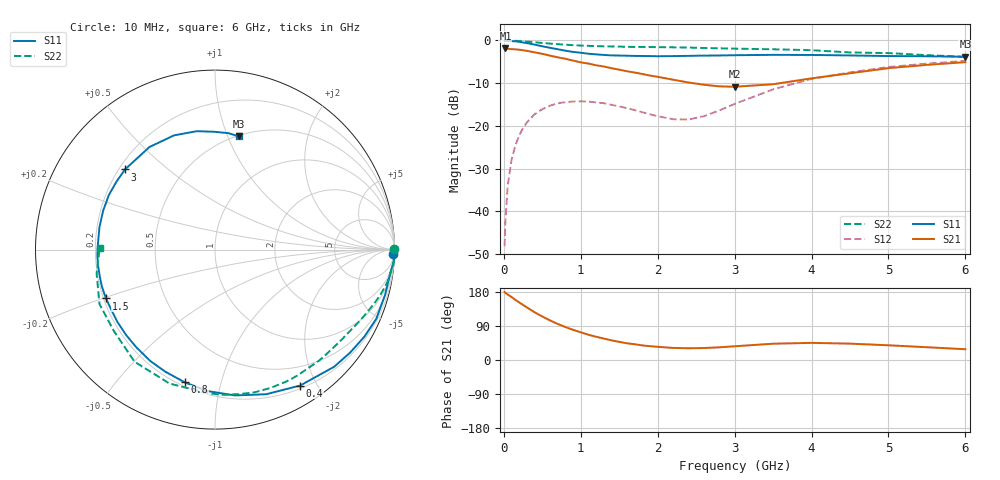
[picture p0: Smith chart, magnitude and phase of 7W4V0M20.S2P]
! Infineon Technologies  Discrete & RF Semiconductors
! BFS17W
! Si NPN RF Bipolar Junction Transistor in SOT323
! VCE = 4 V  IC = 0.2 mA
! Common Emitter S-Parameters:  August  1999
# GHz  S  MA  R  50
!  f  S11  S21  S12  S22
! GHz  MAG  ANG  MAG  ANG  MAG  ANG  MAG  ANG
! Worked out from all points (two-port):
!   36 points, 10 MHz to 6 GHz, reference 50 ohm
!   highest |S21| = -1.87 dB at 20 MHz (marker M1); lowest = -10.8 dB at 3 GHz (marker M2)
!   |S21| within 3 dB of the highest: start of sweep to 937.9 MHz
!   lowest |S11| = -3.8 dB at 6 GHz (marker M3), VSWR 4.63, Z = 25.4 + j54.8 ohm
!   |S11| at or under -10 dB: nowhere
!   |S22| runs from -3.9 to 0.0 dB; largest |S21 - S12| = 0.81
!   S11 on the Smith chart (normalised r, x): 10 MHz: 29, -69; 400 MHz: 0.24, -1.78; 800 MHz: 0.22, -0.77; 1.5 GHz: 0.21, -0.20; 3 GHz: 0.22, +0.36; 6 GHz: 0.51, +1.10
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0.01  0.9897 -1.4  0.797 179.4  0.0039 89.7  0.9999 0.1
0.02  0.9999 -3.3  0.806 177.2  0.0076 91.0  0.9948 -0.8
0.05  0.9852 -7.6  0.8 172.9  0.0199 84.6  0.9984 -2.1
0.1  0.9806 -14.9  0.791 166.2  0.04 81.1  0.9981 -4.3
0.15  0.978 -23.2  0.787 158.8  0.0589 75.3  0.9906 -6.4
0.25  0.9467 -37.3  0.767 145.2  0.0941 66.2  0.9778 -10.3
0.4  0.8938 -57.9  0.726 125.9  0.1367 54.1  0.9528 -15.8
0.6  0.8201 -82.2  0.664 104.4  0.1723 40.8  0.9186 -22.0
0.8  0.7586 -102.8  0.61 87.0  0.1895 30.7  0.8915 -27.8
1.1  0.6989 -128.8  0.536 66.6  0.1924 19.7  0.8646 -35.9
1.5  0.6658 -155.9  0.455 47.9  0.1686 12.5  0.8474 -46.9
1.8  0.6579 -172.6  0.405 38.5  0.1445 13.7  0.8388 -55.9
2.2  0.6558 169.0  0.347 31.9  0.1195 28.1  0.8307 -67.9
2.4  0.6599 160.7  0.322 31.0  0.1186 40.3  0.8255 -74.3
2.6  0.665 152.7  0.303 31.6  0.1297 51.6  0.8163 -80.6
3  0.6715 138.3  0.287 36.2  0.1806 64.8  0.8015 -92.8
3.5  0.6783 122.6  0.307 43.0  0.2676 66.3  0.7883 -108.8
4  0.6762 109.7  0.36 45.2  0.3543 60.4  0.769 -125.6
4.5  0.6675 98.8  0.413 43.2  0.423 52.9  0.7236 -141.2
5  0.6566 90.4  0.474 38.8  0.489 45.5  0.7114 -154.8
5.5  0.653 83.4  0.518 33.7  0.5357 38.2  0.6726 -168.7
6  0.6446 78.2  0.557 28.4  0.5769 31.7  0.6419 179.3
